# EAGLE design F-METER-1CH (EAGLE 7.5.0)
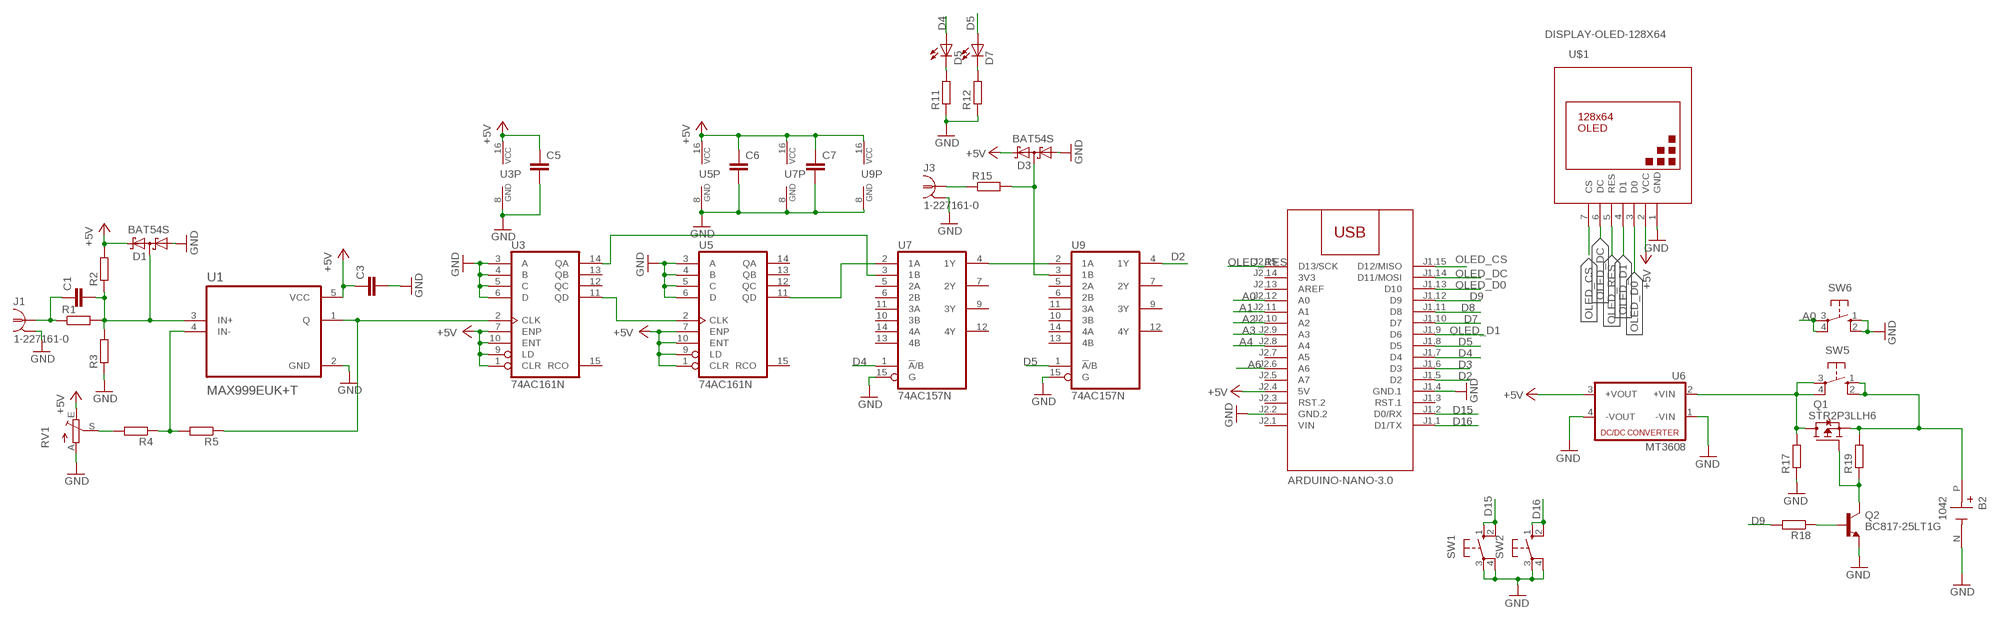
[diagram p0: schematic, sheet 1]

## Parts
ARD1  ARDUINO-NANO-3.0  [ARDUINO-NANO-3.0]
B2  1042  [BAT_1042]
C1  C-EUC1206  [C1206]
C3  C-EUC1206  [C1206]
C5  C-EUC1206  [C1206]
C6  C-EUC1206  [C1206]
C7  C-EUC1206  [C1206]
D1  BAT54S  [SOT23]
D3  BAT54S  [SOT23]
D5  LED3MM  [LED3MM]
D7  LED3MM  [LED3MM]
J1  1-227161-0  [AMP_227161]
J3  1-227161-0  [AMP_227161]
Q1  STR2P3LLH6  [SOT23]
Q2  BC817-25LT1G  [SOT95P237X111-3N]
R1  R-EU_R1206  [R1206]
R2  R-EU_R1206  [R1206]
R3  R-EU_R1206  [R1206]
R4  R-EU_R1206  [R1206]
R5  R-EU_R1206  [R1206]
R11  R-EU_R1206  [R1206]
R12  R-EU_R1206  [R1206]
R15  R-EU_R1206  [R1206]
R17  R-EU_R1206  [R1206]
R18  R-EU_R1206  [R1206]
R19  R-EU_R1206  [R1206]
RV1  TRIM_EU-B64W  [B64W]
SW1  10-XX  [B3F-10XX]
SW2  10-XX  [B3F-10XX]
SW5  10-XX  [B3F-10XX]
SW6  10-XX  [B3F-10XX]
U1  MAX999EUK+T  [SOT95P280X145-5N]
U3  74AC161N  74AC160N  [DIL16]
U5  74AC161N  74AC160N  [DIL16]
U6  MT3608  [MT3608]
U7  74AC157N  [DIL16]
U9  74AC157N  [DIL16]
U$1  DISPLAY-OLED-128X64  [DISPLAY-OLED-128X64]

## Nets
+5V: ARD1.J2.4(5V) C3.1 C5.1 C6.1 C7.1 D1.2(C2) D3.2(C2) R2.2 RV1.E U1.5(VCC) U3.1(CLR) U3.7(ENP) U3.9(LD) U3.10(ENT) U3.16(VCC) U5.1(CLR) U5.7(ENP) U5.9(LD) U5.10(ENT) U5.16(VCC) U6.3(+VOUT) U7.16(VCC) U9.16(VCC) U$1.2(VCC)
A0: ARD1.J2.12(A0) SW6.3(P) SW6.4(P1)
A1: ARD1.J2.11(A1)
A2: ARD1.J2.10(A2)
A3: ARD1.J2.9(A3)
A4: ARD1.J2.8(A4)
A6: ARD1.J2.6(A6)
D2: ARD1.J1.5(D2) U9.4(1Y)
D3: ARD1.J1.6(D3)
D4: ARD1.J1.7(D4) D5.A U7.1(!A!/B)
D5: ARD1.J1.8(D5) D7.A U9.1(!A!/B)
D7: ARD1.J1.10(D7)
D8: ARD1.J1.11(D8)
D9: ARD1.J1.12(D9) R18.2
D15: ARD1.J1.2(D0/RX) SW1.1(S) SW1.2(S1)
D16: ARD1.J1.1(D1/TX) SW2.1(S) SW2.2(S1)
GND: ARD1.J1.4(GND.1) ARD1.J2.2(GND.2) B2.N(NEG) C3.2 C5.2 C6.2 C7.2 D1.1(A1) D3.1(A1) J1.2 J3.2 Q2.2(E) R3.1 R11.1 R12.1 R17.1 RV1.A SW1.3(P) SW1.4(P1) SW2.3(P) SW2.4(P1) SW6.1(S) SW6.2(S1) U1.2(GND) U3.3(A) U3.4(B) U3.5(C) U3.6(D) U3.8(GND) U5.3(A) U5.4(B) U5.5(C) U5.6(D) U5.8(GND) U6.1(-VIN) U6.4(-VOUT) U7.8(GND) U7.15(G) U9.8(GND) U9.15(G) U$1.1(GND)
N$1: C1.1 J1.1 R1.1
N$2: C1.2 D1.3(C1A2) R1.2 R2.1 R3.2 U1.3(IN+)
N$3: R4.2 RV1.S
N$4: R4.1 R5.2 U1.4(IN-)
N$5: R5.1 U1.1(Q) U3.2(CLK)
N$11: U3.11(QD) U5.2(CLK)
N$12: U5.11(QD) U7.2(1A)
N$13: U3.14(QA) U7.3(1B)
N$14: U7.4(1Y) U9.2(1A)
N$15: J3.1 R15.1
N$16: D3.3(C1A2) R15.2 U9.3(1B)
N$17: Q1.2(G) Q2.3(C) R19.1
N$23: B2.P(POS) Q1.3(S) R19.2 SW5.1(S) SW5.2(S1)
N$24: Q2.1(B) R18.1
N$26: Q1.1(D) R17.2 SW5.3(P) SW5.4(P1) U6.2(+VIN)
N$29: D5.K(C) R11.2
N$30: D7.K(C) R12.2
OLED_CS: ARD1.J1.15(D12/MISO) U$1.7(CS)
OLED_D0: ARD1.J1.13(D10) U$1.3(D0)
OLED_D1: ARD1.J1.9(D6) U$1.4(D1)
OLED_DC: ARD1.J1.14(D11/MOSI) U$1.6(DC)
OLED_RES: ARD1.J2.15(D13/SCK) U$1.5(RES)
Unconnected: ARD1.J1.3(RST.1) ARD1.J2.3(RST.2) ARD1.J2.5(A7) ARD1.J2.7(A5) ARD1.J2.13(AREF) U3.12(QC) U3.13(QB) U3.15(RCO) U5.12(QC) U5.13(QB) U5.14(QA) U5.15(RCO) U7.5(2A) U7.6(2B) U7.7(2Y) U7.9(3Y) U7.10(3B) U7.11(3A) U7.12(4Y) U7.13(4B) U7.14(4A) U9.5(2A) U9.6(2B) U9.7(2Y) U9.9(3Y) U9.10(3B) U9.11(3A) U9.12(4Y) U9.13(4B) U9.14(4A)

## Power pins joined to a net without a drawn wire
3V3: ARD1.J2.14(3V3)
VIN: ARD1.J2.1(VIN)

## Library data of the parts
ARD1 = diy-modules:ARDUINO-NANO-3.0: Arduino Nano 3.0 and compatible devices More details available here: https://www.arduino.cc/en/Main/ArduinoBoardNano Click here to find device on ebay.com
B2 = 18650-HOLDER:1042: Check availability; AVAILABILITY: In Stock; CHECK_PRICES: https://www.snapeda.com/parts/1042/Keystone/view-part/?ref=eda; DESCRIPTION: SMT Holder for 18650 Battery; MF: Keystone Electronics Corp.; MP: 1042; PACKAGE: NON STANDARD-5 Keystone; PRICE: None; SNAPEDA_LINK: https://www.snapeda.com/parts/1042/Keystone/view-part/?ref=snap
C1 C3 C5-C7 = rcl:C-EU: CAPACITOR, European symbol
D1 D3 = diode:BAT54S: Schottky Diodes Pin connection corrected 2011-05-04 Source: Fairchild .. BAT54.pdf
D5 D7 = led:LED: LED
J1 J3 = con-coax:?227161*: JACK, RIGHT ANGLE, 50 OHM, PCB, BNC; MF: TYCO ELECTRONICS; MPN: 1-227161; OC_FARNELL: unknown; OC_NEWARK: 33B3200
Q1 = transistor-fet:STR2P3LLH6
Q2 = BC817-25LT1G:BC817-25LT1G: Check availability; AVAILABILITY: In Stock; CHECK_PRICES: https://www.snapeda.com/parts/BC817-25LT1G/Onsemi/view-part/?ref=eda; DESCRIPTION: Transistor NPN 45V 0.5A hfe160 SOT23 | ON Semiconductor BC817-25LT1G; MF: ON Semiconductor; MP: BC817-25LT1G; PACKAGE: SOT-23-3 ON Semiconductor; PRICE: None; PURCHASE-URL: https://www.snapeda.com/api/url_track_click_mouser/?unipart_id=343725&manufacturer=ON Semiconductor&part_name=BC817-25LT1G&search_term=transistor sot23; SNAPEDA_LINK: https://www.snapeda.com/parts/BC817-25LT1G/Onsemi/view-part/?ref=snap
R1-R5 R11 R12 R15 R17-R19 = rcl:R-EU_: RESISTOR, European symbol
RV1 = pot:TRIM_EU-: POTENTIOMETER
SW1 SW2 SW5 SW6 = switch-omron:10-XX: OMRON SWITCH; MPN: B3F-1000; OC_FARNELL: 176432; OC_NEWARK: 36M3542
U1 = MAX999EUK_T:MAX999EUK+T: Check availability; AVAILABILITY: In Stock; CHECK_PRICES: https://www.snapeda.com/parts/MAX999EUK+T/Analog+Devices/view-part/?ref=eda; DESCRIPTION: Single/Dual/Quad, Ultra-High-Speed, +3V/+5V, Beyond-the-Rails Comparators; MF: Analog Devices; MP: MAX999EUK+T; PACKAGE: SOT-23-5 Maxim Integrated; PRICE: None; SNAPEDA_LINK: https://www.snapeda.com/parts/MAX999EUK+T/Analog+Devices/view-part/?ref=snap
U3 U5 = 74xx-eu:74*160: Synchronous 4-bit COUNTER
U6 = dc-dc-converter:MT3608: DC DC Up Converter
U7 U9 = 74xx-eu:74*157: Quadruple 2-line to 1-line data SELECTOR/MULTIPLEXER
U$1 = diy-modules:DISPLAY-OLED-128X64: 128x64 Dot Matrix OLED Module based on SSD1306 chip Variant with SPI interface More details available here: http://www.instructables.com/id/How-to-use-OLED-display-arduino-module/ SSD1306 datasheet: https://cdn-shop.adafruit.com/datasheets/SSD1306.pdf Click here to find device on ebay.com Note: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

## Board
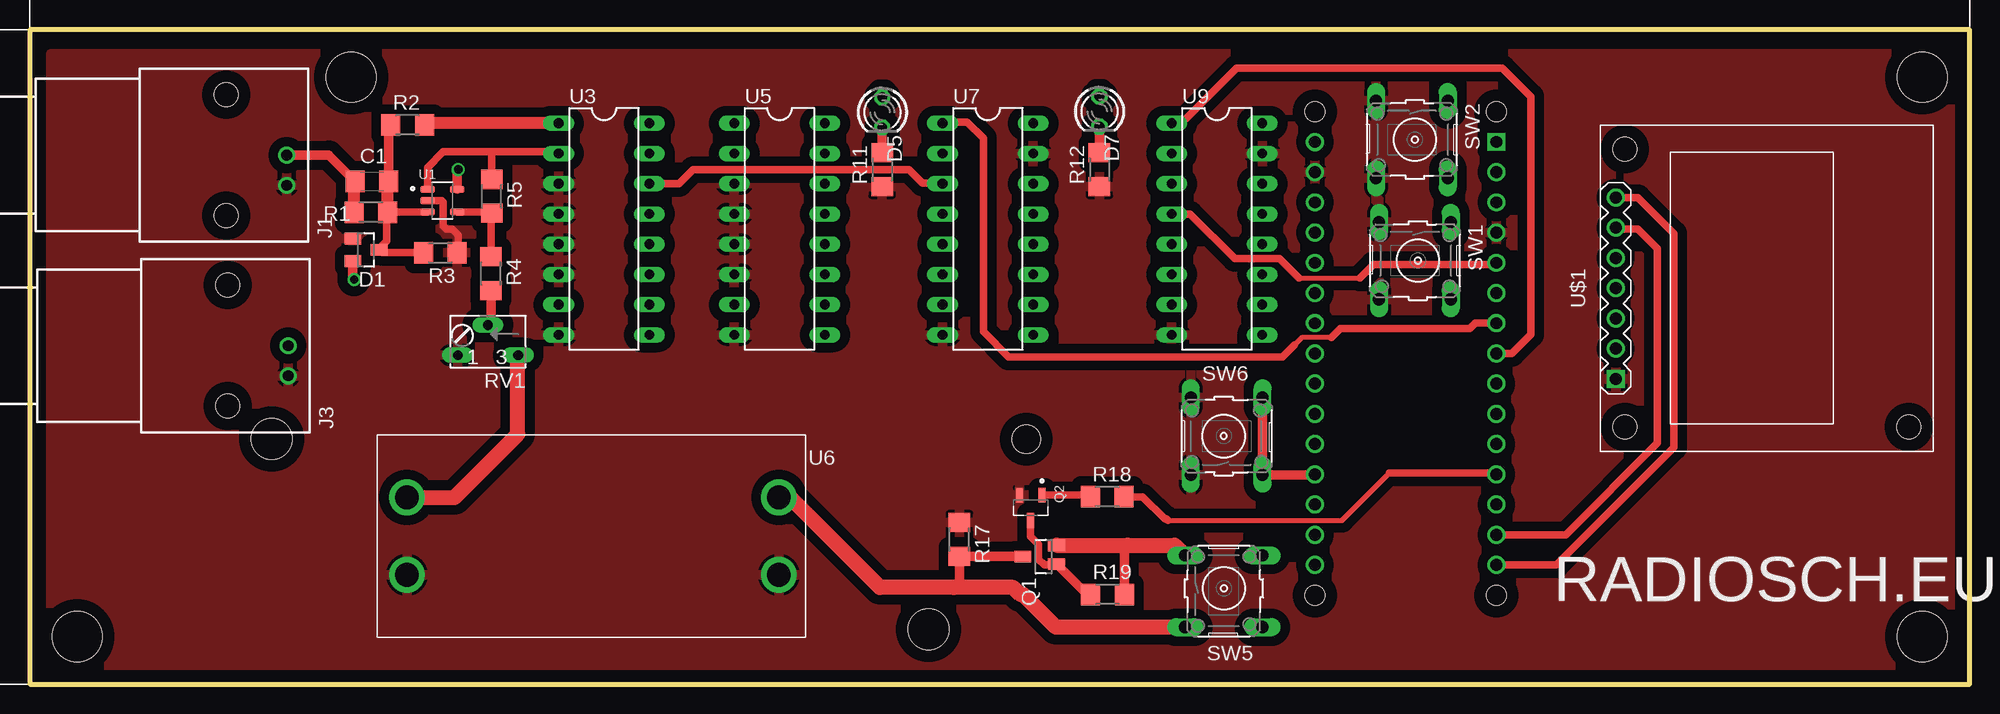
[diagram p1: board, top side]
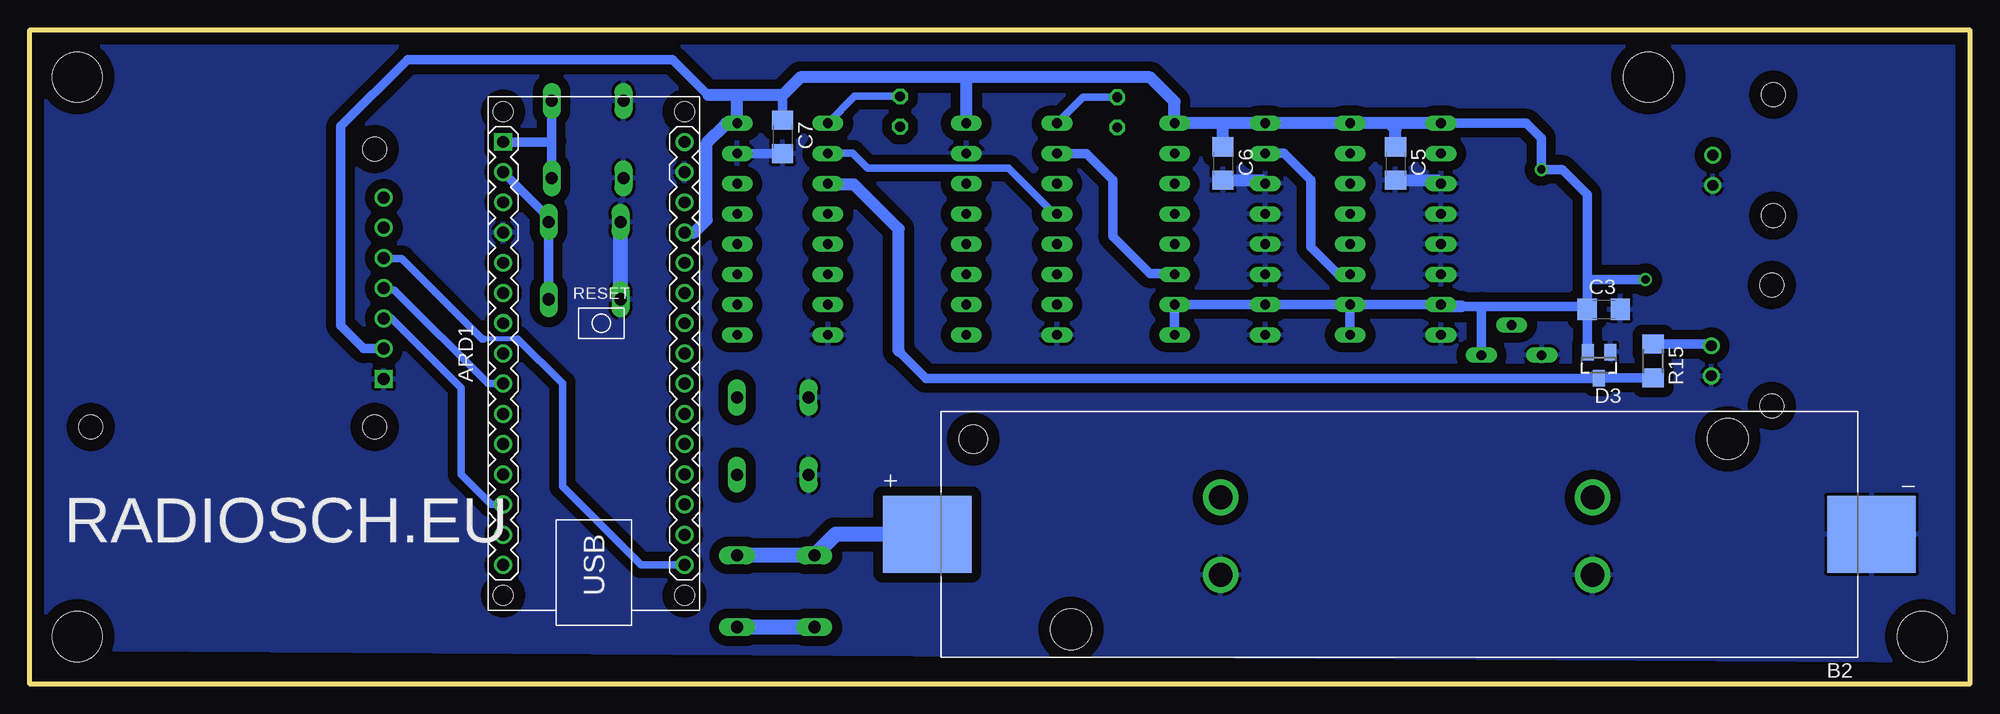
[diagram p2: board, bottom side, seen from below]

Size 163 x 55 mm. Coordinates in mm from the lower left corner, seen from the top.
Outline: 0,0 163,0 163,55 0,55 0,0
Copper layers (1*16): Top 0.035mm / dielectric 1.5mm / Bottom 0.035mm
Design rules "default": minimum track width 10mil, minimum drill 24mil, track to track 8mil, track to pad 8mil, pad to pad 8mil, via to via 8mil, smd to smd 8mil, copper to edge 40mil, drill to drill 8mil, minimum pad ring 10mil, minimum via ring 8mil, stop-mask expansion 4mil, vias tented up to drill 0mil, thermal gap 10mil
Holes 4.2 mm at 4,4 159,51 159,4 27,51

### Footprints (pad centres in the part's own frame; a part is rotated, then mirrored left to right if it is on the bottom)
ARDUINO-NANO-3.0 = drill 1 square: J1.1 17.78,7.62 | drill 1: J1.2 15.24,7.62; J1.3 12.7,7.62; J1.4 10.16,7.62; J1.5 7.62,7.62; J1.6 5.08,7.62; J1.7 2.54,7.62; J1.8 0,7.62; J1.9 -2.54,7.62; J1.10 -5.08,7.62; J1.11 -7.62,7.62; J1.12 -10.16,7.62; J1.13 -12.7,7.62; J1.14 -15.24,7.62; J1.15 -17.78,7.62; J2.1 17.78,-7.62; J2.2 15.24,-7.62; J2.3 12.7,-7.62; J2.4 10.16,-7.62; J2.5 7.62,-7.62; J2.6 5.08,-7.62; J2.7 2.54,-7.62; J2.8 0,-7.62; J2.9 -2.54,-7.62; J2.10 -5.08,-7.62; J2.11 -7.62,-7.62; J2.12 -10.16,-7.62; J2.13 -12.7,-7.62; J2.14 -15.24,-7.62; J2.15 -17.78,-7.62 | hole 1.651: -20.32,7.62; -20.32,-7.62; 20.32,-7.62; 20.32,7.62
BAT_1042 = smd 7.46 x 6.47: N -39.67,0; P 39.67,0 | hole 3.45: 27.6,8; -27.6,-8 | hole 2.39: 35.82,-8
C1206 = smd 1.6 x 1.8: 1 -1.4,0; 2 1.4,0
SOT23 = smd 1 x 1.4: 1 -0.95,-1.1; 2 0.95,-1.1; 3 0,1.1
LED3MM = drill 0.813 octagon: A -1.27,0; K 1.27,0
AMP_227161 = drill 0.9 pad 1.27: 1 0,-5.08; 2 -2.54,-5.08 | hole 2: -5.08,0; 5.08,0
SOT23' = smd 1 x 1.4: 1 0,1.735; 2 -0.632,-1.1; 3 0.95,-1.1
SOT95P237X111-3N = smd 1.23 x 0.6: 1 -1.06,0.95; 2 -1.06,-0.95; 3 1.06,0
R1206 = smd 1.6 x 1.803: 1 -1.422,0; 2 1.422,0
B64W = drill 0.813 long: A 2.54,0; E -2.54,0; S 0,-2.54
B3F-10XX = drill 1.016 long: 1 -3.251,2.761; 2 3.251,2.761; 3 -3.251,-3.261; 4 3.251,-3.261
SOT95P280X145-5N = smd 1.22 x 0.6: 1 -1.245,0.95; 2 -1.245,0; 3 -1.245,-0.95; 4 1.245,-0.95; 5 1.245,0.95
DIL16 = drill 0.813 long: 1 -8.89,-3.81; 2 -6.35,-3.81; 3 -3.81,-3.81; 4 -1.27,-3.81; 5 1.27,-3.81; 6 3.81,-3.81; 7 6.35,-3.81; 8 8.89,-3.81; 9 8.89,3.81; 10 6.35,3.81; 11 3.81,3.81; 12 1.27,3.81; 13 -1.27,3.81; 14 -3.81,3.81; 15 -6.35,3.81; 16 -8.89,3.81
MT3608 = drill 2: 1 2.25,11.75; 2 2.25,5.25; 3 33.5,5.25; 4 33.5,11.75
DISPLAY-OLED-128X64 = drill 1 square: 1 -7.62,12.7 | drill 1: 2 -5.08,12.7; 3 -2.54,12.7; 4 0,12.7; 5 2.54,12.7; 6 5.08,12.7; 7 7.62,12.7 | hole 2: -11.684,11.938; 11.684,11.938; -11.684,-11.938

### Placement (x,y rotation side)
ARD1  115.6,27.79 90 bottom
B2  47.92,12.59 180 bottom
C1  28.75,42.25 0 top
C3  30.75,31.5 0 bottom
C5  48.25,43.75 270 bottom
C6  62.75,43.75 270 bottom
C7  99.75,46 270 bottom
D1  28.25,36.5 270 top
D3  31.15,26.8 180 bottom
D5  71.63,48.06 270 top
D7  89.88,48.12 270 top
J1  16.52,44.47 90 top
J3  16.64,28.45 90 top
Q1  STR2P3LLH6  [SOT23']  85.17,10.72 90 top
Q2  84.09,14.82 270 top
R1  28.66,39.66 0 top
R2  31.75,47 0 top
R3  34.5,36.25 180 top
R4  38.75,34.5 270 top
R5  38.81,41 270 top
R11  71.62,43.25 90 top
R12  89.88,43.25 90 top
R15  26.6,27.15 270 bottom
R17  78.1,12.15 270 top
R18  90.53,15.75 0 top
R19  90.56,7.53 0 top
RV1  38.5,27.64 180 top
SW1  116.63,35.59 270 top
SW2  116.38,45.77 270 top
SW5  100.33,8.05 0 top
SW6  100.32,20.84 90 top
U1  34.67,40.64 0 top
U3  48.25,38.25 270 top
U5  63,38.25 270 top
U6  65.19,20.94 180 top
U7  80.5,38.25 270 top
U9  99.75,38.25 270 top
U$1  145.95,33.28 90 top

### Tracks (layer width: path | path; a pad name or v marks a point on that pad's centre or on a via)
+5V  (via drill 0.7)
  Top 0.813: U1.5 35.91,43.17 v36,43.25 | D1.2 27.15,34.1 v27.25,34
  Top 1.016: U3.1 33.31,47.14 R2.2
  Top 1.27: U6.3 35.69,15.69 41,21 41,27.6 RV1.E
  Bottom 0.813: U3.7 U3.10 52.62,31.9 | 52.62,31.9 U5.7 U5.10 U5.9 | U3.9 52.06,31.33 52.62,31.9 | C7.1 99.75,49.5 | C3.1 32.15,27.95 D3.2 | U3.1 37.25,47.14 36,45.89 v36,43.25 34.25,43.25 32.15,41.15 32.15,34 | C3.1 32.15,34 | v27.25,34 32.15,34 | 42.75,31.75 41,31.75 | 41,31.75 32.4,31.75 C3.1 | RV1.E 41.04,31.71 41,31.75 | U$1.2 134.94,28.2 136.88,30.12 136.88,46.88 131.25,52.5 109,52.5 106,49.5
  Bottom 1.016: U3.1 48.75,47.14 | 48.75,47.14 U3.16 U5.1 62.5,47.14 | 62.5,47.14 U5.16 | C5.1 48.25,46.64 48.75,47.14 | U5.16 66.81,47.31 | 103.5,49.5 99.75,49.5 98.25,51 84.5,51 | 103.5,49.5 106,49.5 | 103.5,49.5 103.56,49.44 U9.16 103.58,47.12 104.5,47.12 106.12,45.5 106.12,39 107.17,37.95 ARD1.J2.4 | C6.1 62.75,46.89 62.5,47.14 | U5.16 66.81,48.94 68.88,51 84.5,51 | U7.16 84.31,50.81 84.5,51 | 42.75,31.75 44.29,31.75 U3.7
A0
  Top 0.813: SW6.4 SW6.3 107.94,17.59 ARD1.J2.12
D2
  Top 0.406: 106.62,34.12 111.75,34.12
  Top 0.61: U9.4 97.48,39.52 101.25,35.75 105,35.75 106.62,34.12 | 111.75,34.12 112.88,35.25 123.06,35.25 ARD1.J1.5
D4
  Top 0.406: 109.38,29.12 106.88,29.12 106.25,28.5
  Top 0.61: ARD1.J1.7 121.45,30.33 121,29.88 110.12,29.88 109.38,29.12 | 106.25,28.5 105.25,27.5 82.25,27.5 80.12,29.62 80.12,45.88 78.75,47.25 76.8,47.25 U7.1
  Bottom 0.61: D5.A 74.5,49.33 U7.1
D5
  Top 0.61: U9.1 96.77,47.14 101.38,51.75 123.75,51.75 126.12,49.38 126.12,29.38 124.54,27.79 ARD1.J1.8
  Bottom 0.61: D7.A 93.69,49.39 U9.1
D9
  Top 0.406: 95.62,13.75 110.25,13.75 114.25,17.75
  Top 0.61: R18.2 93.5,15.75 95.38,13.88 95.5,13.88 95.62,13.75 | 114.25,17.75 123.1,17.75 ARD1.J1.12
D15
  Bottom 0.813: SW1.2 SW1.1 119.39,39.2 ARD1.J1.2
D16
  Bottom 0.813: SW2.2 119.14,45.62 | 119.14,45.62 SW2.1 | ARD1.J1.1 119.2,45.57 119.14,45.62
GND
  Top 0.61: U1.2 34.61,40.64 34.75,40.5 34.75,38.5 35,38.25 35.5,38.25 36,37.75 36,36.33 R3.1
  Bottom 0.813: C7.2 U9.15
  Bottom 1.016: C5.2 44.73,42.35 U3.3 | C6.2 59.48,42.35 U5.3
  Bottom 1.27: 113.42,32.29 SW1.4 SW1.3
  pour Bottom (isolate 0.813): 1,56 163,57 163,3 1,2
  pour Top (isolate 0.813): 1.75,53 162.5,53 162.5,0.75 1.75,0.75 1.75,52.75
N$1
  Top 0.813: J1.1 25.14,44.47 C1.1
  Top 1.016: R1.1 27.24,42.14 C1.1
N$2
  Top 0.61: U1.3 33.39,39.66 R1.2 30,39.58 30,37.25 29.35,36.6 D1.3 29.6,36.25 R3.2
  Top 0.813: C1.2 30.15,46.57 R2.1
  Top 1.016: R1.2 30.08,42.18 C1.2
N$3
  Top 0.813: R4.2 38.75,30.43 RV1.S
N$4
  Top 0.61: R4.1 38.75,39.52 R5.2 38.7,39.69 U1.4
N$5
  Top 0.61: U1.1 33.42,43.42 34.75,44.75 38.75,44.75 | 38.75,44.75 44.29,44.75 U3.2 | R5.1 38.81,44.69 38.75,44.75
N$11
  Bottom 0.813: U3.11 53.06,34.44 55.38,36.75 55.38,42.38 57.62,44.62 59.16,44.62 U5.2
N$12
  Bottom 0.813: U7.2 74.22,44.6 72,42.38 72,37.62 68.88,34.5 66.87,34.5 U5.11
N$13
  Top 0.61: U3.14 54.56,42.06 55.75,43.25 73.88,43.25 75,42.12 76.62,42.12 U7.3
N$14
  Bottom 0.61: U7.4 76.89,39.52 80.75,43.38 92.62,43.38 93.88,44.62 95.92,44.62 U9.2
N$15
  Bottom 0.813: R15.1 21.85,28.57 J3.1
N$16
  Bottom 0.813: R15.2 31.12,25.73 D3.3 87.7,25.7 90,28
  Bottom 1.016: 90,28 90,38.25 93.75,42 95.88,42 U9.3
N$17
  Top 0.61: Q1.2 86.19,10 85.25,10 84.75,10.5 84.75,11.75 84.09,12.41 Q2.3
  Top 0.813: R19.1 88.82,7.53 Q1.2
N$23
  Top 0.813: R19.2 91.98,11.39 92.25,11.66
  Top 1.27: Q1.3 92.25,11.66 96.22,11.66 SW5.1
  Bottom 1.27: B2.P 95.29,12.59 SW5.1 SW5.2
N$24
  Top 0.61: Q2.1 88.98,15.88 R18.1
N$26
  Top 0.813: 77.62,8.12 78.1,8.6 R17.2 78.11,10.72 Q1.1
  Top 1.27: U6.2 63.88,15.69 71.44,8.12 77.62,8.12 82.62,8.12 83.25,7.5 83.5,7.5 86.21,4.79 SW5.3
  Bottom 1.27: SW5.3 SW5.4
N$29
  Top 0.813: R11.2 D5.K
N$30
  Top 0.813: R12.2 D7.K
OLED_CS
  Top 0.61: ARD1.J1.15 128.26,10.01 138.12,19.88 138.12,37.88 135.12,40.88 133.27,40.88 U$1.7
OLED_D0
  Bottom 0.61: ARD1.J1.13 124.22,15.09 126.75,17.62 126.75,24.88 132.62,30.75 133.24,30.75 U$1.3
OLED_D1
  Bottom 0.61: ARD1.J1.9 124.5,25.25 132.38,33.12 133.1,33.12 U$1.4
OLED_DC
  Top 0.61: ARD1.J1.14 129.05,12.55 136.75,20.25 136.75,36.62 135.12,38.25 133.36,38.25 U$1.6
OLED_RES
  Bottom 0.406: 122,29 124.88,29
  Bottom 0.61: ARD1.J2.15 111.64,10.01 118.25,16.62 118.25,25.25 122,29 | 124.88,29 125,29 131.75,35.75 133.19,35.75 U$1.5

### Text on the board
tPlace: RADIOSCH.EU
bPlace: RADIOSCH.EU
